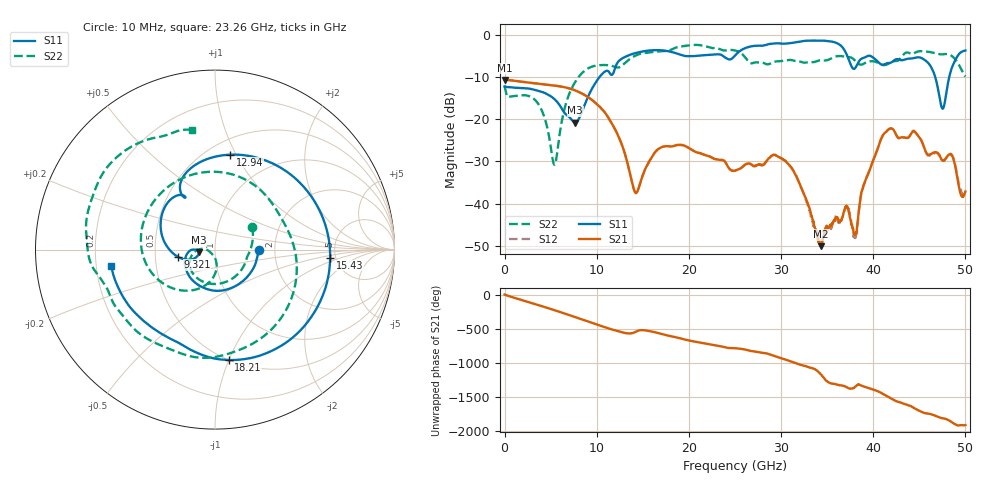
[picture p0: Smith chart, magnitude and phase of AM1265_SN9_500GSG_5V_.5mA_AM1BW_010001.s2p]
!Keysight Technologies,N5245B,MY58422270,A.16.20.02
!Date: Thursday, March 05, 2026 00:53:07
!Correction: S11(C  2-Port  )
!S21(C  2-Port  )
!S12(C  2-Port  )
!S22(C  2-Port  )
!S2P File: Measurements: S11, S21, S12, S22:
# Hz S  dB  R 50
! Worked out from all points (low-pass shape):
!   3201 points, 10 MHz to 50 GHz, reference 50 ohm
!   highest |S21| = -10.71 dB at 25.62 MHz (marker M1); lowest = -50.1 dB at 34.33 GHz (marker M2)
!   |S21| within 3 dB of the highest: start of sweep to 8.191 GHz
!   lowest |S11| = -20.8 dB at 7.665 GHz (marker M3), VSWR 1.20, Z = 41.8 - j1.18 ohm
!   |S11| at or under -10 dB: start of sweep to 10.32 GHz; 46.72 GHz to 48.25 GHz (1.528 GHz wide, 3.22 % of centre)
!   |S22| runs from -30.8 to -2.4 dB; largest |S21 - S12| = 0.0022
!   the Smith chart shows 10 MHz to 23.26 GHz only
!   S11 on the Smith chart (normalised r, x): 10 MHz: 1.64, -0.01; 9.321 GHz: 0.65, -0.05; 12.94 GHz: 0.64, +0.95; 15.43 GHz: 4.50, -0.68; 18.21 GHz: 0.50, -1.00; 23.26 GHz: 0.26, -0.07
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1e7  -12.26 -0.4  -10.71 3.5  -10.65 3.7  -12.28 30.9
2.562188e7  -12.27 -0.8  -10.71 2.8  -10.66 3.0  -12.43 28.7
3.634275e9  -13.27 -117.0  -11.61 -149.8  -11.61 -149.8  -16.31 -156.2
5.415169e9  -15.27 -163.7  -12.08 134.7  -12.07 134.8  -30.81 -135.5
7.664719e9  -20.84 -171.1  -13.21 32.6  -13.21 32.7  -11.22 -123.6
8.352081e9  -18.51 -157.3  -13.89 0.7  -13.88 0.8  -9.23 -147.0
9.320638e9  -13.50 -169.2  -15.18 -44.2  -15.19 -44.2  -7.72 177.8
1.125775e10  -8.66 125.5  -19.62 -132.2  -19.62 -132.4  -7.25 90.3
1.294491e10  -5.42 80.8  -27.40 163.6  -27.40 163.8  -6.95 -3.0
1.542879e10  -3.83 -4.0  -31.07 -165.7  -31.10 -165.9  -4.32 -112.5
1.667854e10  -3.67 -41.9  -27.10 158.2  -27.13 158.3  -4.00 -143.0
1.820948e10  -4.15 -83.0  -26.46 108.0  -26.39 107.8  -3.45 -168.6
2.325535e10  -4.67 -171.1  -29.62 -30.0  -29.54 -30.1  -3.36 100.8
2.5005e10  -4.96 175.4  -32.20 -63.3  -32.19 -63.8  -3.75 70.1
2.951972e10  -2.06 96.5  -28.66 171.0  -28.68 171.0  -6.33 -18.1
3.334708e10  -1.42 35.7  -43.17 6.1  -44.04 1.6  -6.54 -132.7
3.433126e10  -1.39 18.5  -50.08 -88.3  -49.68 -89.5  -6.06 -154.7
3.808051e10  -7.81 -24.6  -47.31 96.2  -48.11 96.9  -6.30 133.1
4.167354e10  -6.73 -54.4  -22.45 -59.7  -22.38 -59.7  -6.89 112.4
4.512598e10  -5.44 -100.6  -24.72 90.9  -24.71 89.9  -3.91 74.7
4.773483e10  -16.39 65.3  -29.75 -15.9  -29.68 -16.6  -4.61 40.5
5e10  -3.75 -71.1  -37.15 -110.7  -38.14 -117.1  -9.92 8.5
